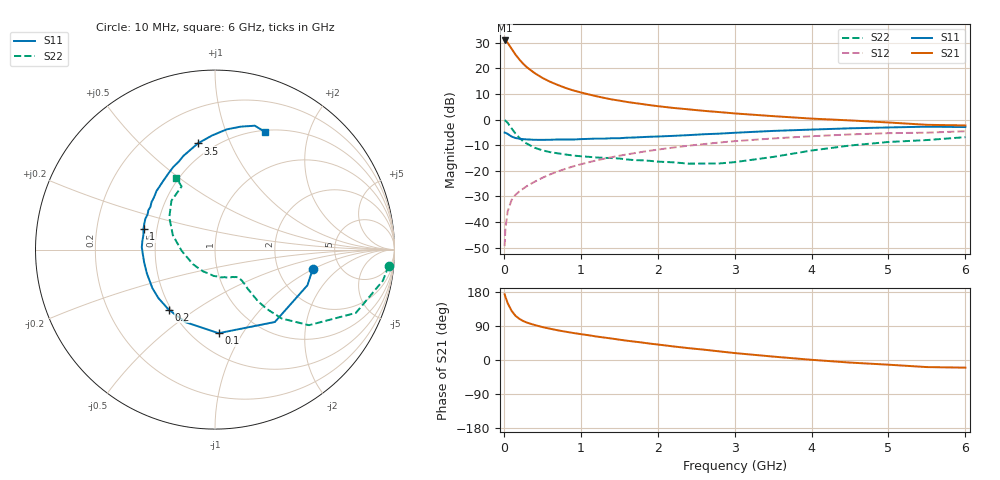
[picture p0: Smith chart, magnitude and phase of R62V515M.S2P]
! SIEMENS Small Signal Semiconductors
! BFR193
! Si NPN RF Bipolar Junction Transistor in SOT23
! VCE = 2.5 V  IC = 15 mA
! Common Emitter S-Parameters:  May  1996
# GHz  S  MA  R  50
!  f  S11  S21  S12  S22
! GHz  MAG  ANG  MAG  ANG  MAG  ANG  MAG  ANG
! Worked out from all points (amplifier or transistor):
!   36 points, 10 MHz to 6 GHz, reference 50 ohm
!   highest |S21| = 30.8 dB at 10 MHz (marker M1)
!   |S21| within 3 dB of that: start of sweep to 95.64 MHz
!   unconditionally stable (mu >= 1): 626.1 MHz to 1.998 GHz
!   at 250 MHz: K = 0.77, MSG = 24.4 dB, |S12| = -27.0 dB
!   at 1.4 GHz: K = 1.03, MAG = 10.2 dB, |S12| = -14.7 dB
!   at 6 GHz: K = 0.95, MSG = 1.1 dB, |S12| = -4.6 dB
!   S11 on the Smith chart (normalised r, x): 10 MHz: 3.17, -0.97; 100 MHz: 0.67, -0.79; 200 MHz: 0.48, -0.39; 1 GHz: 0.42, +0.12; 3.5 GHz: 0.41, +0.76; 6 GHz: 0.52, +1.38
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0.01  0.5554 -11.0  34.71 173.6  0.0034 87.4  0.9718 -5.3
0.02  0.552 -21.1  34.18 167.0  0.0072 78.5  0.9513 -10.5
0.05  0.5234 -50.4  31.16 150.0  0.0163 73.3  0.8604 -24.2
0.1  0.4662 -87.5  24.02 130.0  0.0268 62.7  0.6721 -38.8
0.15  0.4364 -112.1  18.55 117.0  0.0339 59.3  0.5347 -45.9
0.2  0.4224 -127.7  14.9 108.9  0.0395 59.7  0.4413 -48.8
0.25  0.4152 -139.3  12.26 103.0  0.0447 60.1  0.3777 -50.2
0.3  0.4097 -148.3  10.41 98.7  0.0504 61.4  0.338 -50.2
0.4  0.4022 -160.6  8.032 92.3  0.0612 63.7  0.2819 -50.1
0.5  0.4012 -169.6  6.483 87.0  0.073 65.2  0.2508 -49.3
0.6  0.4028 -176.3  5.45 82.6  0.085 66.0  0.2315 -49.1
0.7  0.408 178.2  4.72 78.4  0.0971 66.2  0.2194 -49.4
0.8  0.4075 173.0  4.135 74.8  0.1091 66.1  0.2082 -50.4
1  0.4148 163.8  3.371 68.3  0.1339 65.7  0.1923 -52.4
1.1  0.4193 160.0  3.093 65.4  0.1464 65.0  0.1875 -54.9
1.3  0.4236 152.5  2.647 59.4  0.1715 63.3  0.179 -58.9
1.6  0.4419 143.1  2.199 50.9  0.2087 60.2  0.1666 -68.2
2.2  0.4798 126.8  1.683 35.9  0.2839 52.9  0.1465 -93.4
3.5  0.5992 99.2  1.163 9.0  0.4274 33.6  0.1864 -178.1
4.5  0.6732 84.4  0.96 -6.8  0.5119 19.1  0.3113 144.8
5.5  0.725 72.2  0.788 -18.7  0.5536 4.4  0.3978 117.9
6  0.7126 66.8  0.767 -20.2  0.5908 0.0  0.4528 118.3
